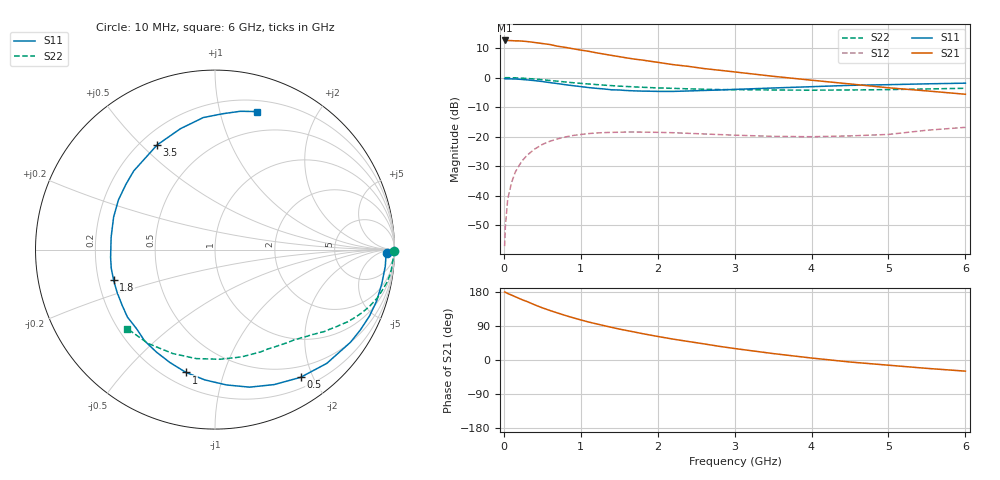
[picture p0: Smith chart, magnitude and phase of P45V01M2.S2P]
! SIEMENS Small Signal Semiconductors
! BFP182
! Si NPN RF Bipolar Junction Transistor in SOT143
! VCE = 5 V  IC = 1.2 mA
! Common Emitter S-Parameters:  March  1996
# GHz  S  MA  R  50
!  f  S11  S21  S12  S22
! GHz  MAG  ANG  MAG  ANG  MAG  ANG  MAG  ANG
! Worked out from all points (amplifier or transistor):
!   36 points, 10 MHz to 6 GHz, reference 50 ohm
!   highest |S21| = 12.6 dB at 10 MHz (marker M1)
!   |S21| within 3 dB of that: start of sweep to 941.6 MHz
!   unconditionally stable (mu >= 1): 2.556 GHz to end of sweep
!   at 250 MHz: K = 0.10, MSG = 20.1 dB, |S12| = -27.8 dB
!   at 1.4 GHz: K = 0.56, MSG = 13.0 dB, |S12| = -18.6 dB
!   at 6 GHz: K = 1.04, MAG = 4.4 dB, |S12| = -16.9 dB
!   S11 on the Smith chart (normalised r, x): 10 MHz: 38, -19; 500 MHz: 0.34, -1.82; 1 GHz: 0.28, -0.75; 1.8 GHz: 0.26, -0.14; 3.5 GHz: 0.27, +0.56; 6 GHz: 0.30, +1.30
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0.01  0.9593 -1.2  4.247 179.4  0.0014 84.6  0.9979 -0.4
0.02  0.9533 -2.2  4.236 178.8  0.003 80.9  0.9932 -0.9
0.05  0.9532 -5.6  4.24 175.6  0.0087 88.2  0.9966 -2.2
0.1  0.9486 -11.5  4.218 171.3  0.0167 82.5  0.9904 -4.3
0.15  0.9453 -17.6  4.177 166.9  0.0253 78.6  0.9892 -6.5
0.25  0.9254 -28.9  4.128 158.1  0.0406 72.4  0.9744 -10.8
0.3  0.9144 -34.4  4.075 154.4  0.0481 68.4  0.9648 -12.7
0.4  0.8887 -45.5  3.924 145.6  0.0616 62.5  0.9442 -16.5
0.5  0.8566 -56.2  3.768 137.7  0.0737 56.3  0.9189 -19.9
0.6  0.8212 -66.3  3.622 130.6  0.0837 50.6  0.8928 -23.1
0.8  0.7569 -85.1  3.242 117.5  0.0987 40.8  0.8423 -28.5
1  0.7033 -103.3  2.916 105.8  0.1087 32.7  0.7977 -32.8
1.1  0.6773 -111.8  2.787 100.3  0.1126 29.3  0.7785 -34.7
1.4  0.6206 -134.8  2.372 86.2  0.1181 20.1  0.7305 -40.0
1.5  0.6159 -142.4  2.26 81.7  0.1187 18.0  0.7162 -41.5
1.8  0.5899 -163.3  1.978 69.6  0.1193 12.3  0.6855 -45.9
2.2  0.5828 173.2  1.655 55.1  0.1165 6.4  0.6569 -52.1
2.8  0.6154 143.7  1.332 36.1  0.1084 2.4  0.6269 -62.1
3.5  0.6661 119.0  1.051 17.0  0.1011 2.8  0.616 -76.0
4.5  0.7384 95.1  0.78 -5.3  0.1029 10.7  0.6162 -99.7
5.5  0.7832 79.7  0.594 -22.1  0.1284 17.3  0.642 -125.4
6  0.8039 73.1  0.522 -29.4  0.1437 15.6  0.6585 -138.1
